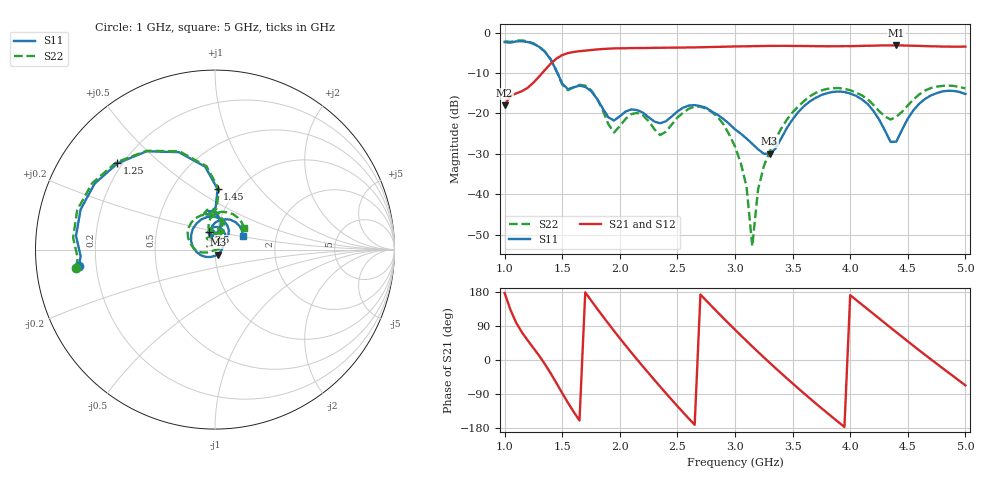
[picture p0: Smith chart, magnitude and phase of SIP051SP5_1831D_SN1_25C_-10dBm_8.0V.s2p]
# GHz  S  dB  R  50
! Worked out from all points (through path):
!   81 points, 1 GHz to 5 GHz, reference 50 ohm
!   highest |S21| = -3.17 dB at 4.4 GHz (marker M1); lowest = -18.0 dB at 1 GHz (marker M2)
!   lowest |S11| = -30.0 dB at 3.3 GHz (marker M3), VSWR 1.07, Z = 51.4 - j2.88 ohm
!   |S11| at or under -10 dB: 1.459 GHz to end of sweep
!   |S22| runs from -52.8 to -2.0 dB; largest |S21 - S12| = 0.0031
!   S11 on the Smith chart (normalised r, x): 1 GHz: 0.14, -0.06; 1.25 GHz: 0.18, +0.37; 1.45 GHz: 0.82, +0.62; 2.5 GHz: 0.92, +0.19; 5 GHz: 1.35, +0.21
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1  -2.36 -173.3  -17.98 176.9  -17.96 177.1  -2.15 -172.6
1.25  -2.79 138.5  -12.39 31.7  -12.39 31.9  -2.68 138.6
1.45  -9.44 87.5  -6.43 -61.0  -6.42 -61.0  -9.48 86.1
1.55  -14.02 101.3  -5.07 -112.9  -5.06 -112.8  -14.27 101.5
1.7  -13.42 93.6  -4.47 178.5  -4.46 178.5  -13.12 92.0
1.95  -21.74 100.0  -3.91 76.7  -3.92 76.8  -24.69 97.4
2.15  -19.14 98.3  -3.83 1.3  -3.83 1.4  -19.86 99.7
2.35  -22.43 102.7  -3.76 -70.1  -3.77 -70.1  -25.33 102.4
2.5  -19.50 109.1  -3.73 -121.7  -3.73 -121.7  -21.02 123.1
2.75  -18.62 66.7  -3.61 156.8  -3.61 157.0  -18.81 74.3
3  -23.93 33.7  -3.44 80.0  -3.43 80.1  -28.17 23.7
3.1  -26.20 20.5  -3.40 50.3  -3.38 50.3  -38.01 2.2
3.15  -27.51 10.8  -3.37 35.7  -3.35 35.8  -52.80 -76.8
3.2  -28.84 -4.5  -3.35 21.3  -3.34 21.5  -38.81 -150.4
3.3  -29.96 -61.8  -3.29 -7.0  -3.30 -6.9  -29.52 -157.9
3.5  -21.46 -157.9  -3.31 -61.8  -3.30 -61.9  -19.71 -176.8
3.7  -16.14 148.3  -3.37 -114.3  -3.37 -114.2  -14.92 148.3
4  -15.07 82.0  -3.37 171.1  -3.37 171.1  -14.26 95.1
4.35  -27.00 60.1  -3.19 85.5  -3.19 85.5  -21.49 88.5
4.4  -26.98 90.7  -3.17 73.4  -3.17 73.3  -20.82 99.7
4.7  -15.55 80.7  -3.39 1.9  -3.37 2.0  -13.71 86.9
5  -15.19 25.6  -3.47 -67.0  -3.48 -66.8  -13.81 37.1
